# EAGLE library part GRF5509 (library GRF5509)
RF Amplifier High Efficiency, 5.0Watt PA/Saturated PA, OP1dB >34.0 dBm, 900 MHz ISM; 0.7 - 01.8 GHz Source: Datasheet
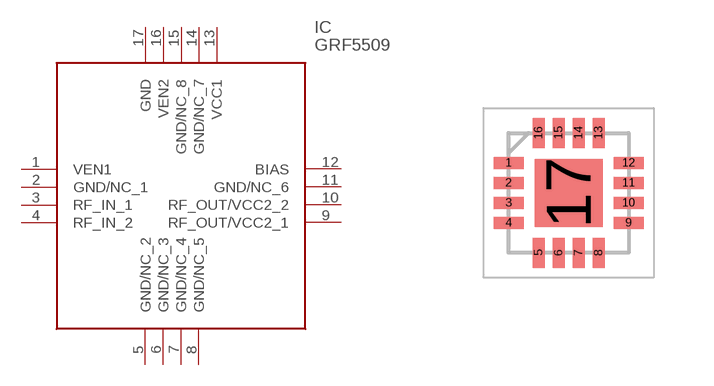
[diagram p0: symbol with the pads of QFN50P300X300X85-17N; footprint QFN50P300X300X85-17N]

Designator prefix IC

## GRF5509 (Description: RF Amplifier High Efficiency, 5.0Watt PA/Saturated PA, OP1dB >34.0 dBm, 900 MHz ISM; 0.7 - 01.8 GHz; Height: 0.85mm; Manufacturer_Name: Guerrilla RF; Manufacturer_Part_Number: GRF5509; Mouser_Part_Number: 459-GRF5509; Mouser_Price-Stock: https://www.mouser.co.uk/ProductDetail/Guerrilla-RF/GRF5509?qs=hWgE7mdIu5TgcXKIFMHrBQ%3D%3D)  [QFN50P300X300X85-17N]
1  VEN1
2  GND/NC_1
3  RF_IN_1
4  RF_IN_2
5  GND/NC_2
6  GND/NC_3
7  GND/NC_4
8  GND/NC_5
9  RF_OUT/VCC2_1
10  RF_OUT/VCC2_2
11  GND/NC_6
12  BIAS
13  VCC1
14  GND/NC_7
15  GND/NC_8
16  VEN2
17  GND

## Footprint QFN50P300X300X85-17N (pad centres in mm)
QFN-16A
smd 0.75 x 0.3: 1 -1.5,0.75; 2 -1.5,0.25; 3 -1.5,-0.25; 4 -1.5,-0.75; 9 1.5,-0.75; 10 1.5,-0.25; 11 1.5,0.25; 12 1.5,0.75
smd 0.3 x 0.75: 5 -0.75,-1.5; 6 -0.25,-1.5; 7 0.25,-1.5; 8 0.75,-1.5; 13 0.75,1.5; 14 0.25,1.5; 15 -0.25,1.5; 16 -0.75,1.5
smd 1.7 x 1.7: 17 0,0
